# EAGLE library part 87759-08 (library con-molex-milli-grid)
HEADER
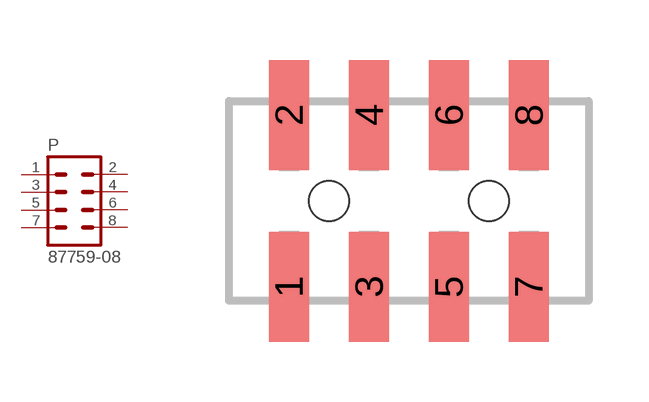
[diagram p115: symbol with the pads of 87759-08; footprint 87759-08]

Designator prefix P

## 87759-08  [87759-08]
1  1  pas
2  2  pas
3  3  pas
4  4  pas
5  5  pas
6  6  pas
7  7  pas
8  8  pas

## Footprint 87759-08 (pad centres in mm)
HEADER SMD Dual Row, Vertical
smd 1 x 2.75: 1 -3,-2.15; 2 -3,2.15; 3 -1,-2.15; 4 -1,2.15; 5 1,-2.15; 6 1,2.15; 7 3,-2.15; 8 3,2.15
hole 1 at -2,0
hole 1 at 2,0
